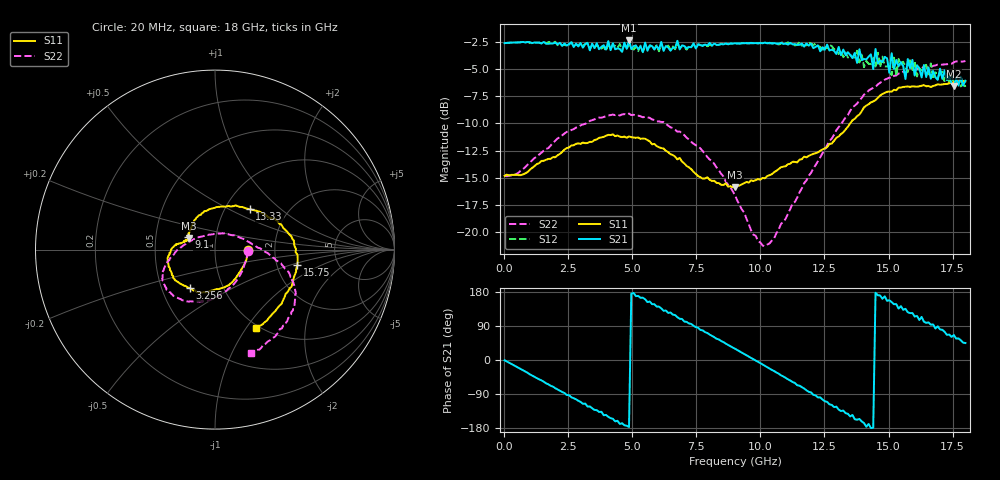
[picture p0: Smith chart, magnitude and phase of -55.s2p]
!Agilent Technologies,N5230A,US43500223,A.07.50.48
!Agilent N5230A: A.07.50.48
!Date: Saturday, January 16, 2016 19:57:11
!Correction: S11(Full 2 Port(1,2))
!S21(Full 2 Port(1,2))
!S12(Full 2 Port(1,2))
!S22(Full 2 Port(1,2))
!S2P File: Measurements: S11, S21, S12, S22:
# Hz S  dB  R 50
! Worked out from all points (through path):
!   201 points, 20 MHz to 18 GHz, reference 50 ohm
!   highest |S21| = -2.38 dB at 4.875 GHz (marker M1); lowest = -6.6 dB at 17.55 GHz (marker M2)
!   group delay of S21, straight-line fit = 105 ps
!   lowest |S11| = -15.9 dB at 9.01 GHz (marker M3), VSWR 1.38, Z = 36.9 + j4.94 ohm
!   |S11| at or under -10 dB: start of sweep to 13.51 GHz
!   |S22| runs from -21.3 to -4.3 dB; largest |S21 - S12| = 0.15
!   S11 on the Smith chart (normalised r, x): 20 MHz: 1.44, -0.01; 3.256 GHz: 0.69, -0.32; 9.1 GHz: 0.74, +0.10; 13.33 GHz: 1.30, +0.64; 15.75 GHz: 2.61, -0.58; 18 GHz: 0.96, -1.11
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2e7  -14.82 -1.6  -2.63 -0.7  -2.62 -0.7  -14.82 -1.9
9.19e8  -14.47 -47.3  -2.52 -33.8  -2.53 -34.1  -13.78 -50.1
1.818e9  -13.26 -81.0  -2.66 -68.1  -2.58 -68.9  -12.02 -82.4
3.0766e9  -11.76 -117.8  -3.04 -115.6  -2.91 -114.9  -10.10 -111.9
3.2564e9  -11.80 -123.5  -2.62 -122.9  -2.59 -122.1  -9.93 -115.4
4.8746e9  -11.20 -160.0  -2.38 -176.7  -2.74 -177.3  -9.10 -140.6
6.0433e9  -12.20 -178.9  -3.20 140.9  -3.38 139.1  -9.82 -155.4
7.3918e9  -14.44 168.7  -2.65 90.3  -2.75 90.8  -11.87 -169.0
9.01e9  -15.89 156.1  -2.65 29.8  -2.67 29.4  -16.60 162.2
9.0999e9  -15.76 155.3  -2.66 26.2  -2.64 25.7  -17.09 158.8
1.05383e10  -14.48 131.5  -2.63 -29.2  -2.74 -30.3  -20.55 71.4
1.20666e10  -12.79 95.0  -3.09 -91.9  -2.81 -90.2  -14.13 11.8
1.33252e10  -10.56 49.2  -3.73 -140.3  -3.47 -139.4  -9.45 -8.6
1.4404e10  -7.98 17.7  -5.01 -178.5  -3.98 179.3  -6.74 -21.6
1.44939e10  -7.86 16.2  -3.16 177.6  -4.78 179.8  -6.64 -21.8
1.50333e10  -7.07 4.3  -5.36 157.8  -4.79 152.2  -5.80 -28.7
1.56626e10  -6.64 -8.9  -5.92 135.1  -4.75 129.8  -5.30 -37.0
1.57525e10  -6.61 -10.7  -4.09 126.0  -5.28 130.5  -5.19 -37.8
1.58424e10  -6.65 -13.4  -4.93 123.7  -4.08 118.7  -5.20 -39.3
1.66515e10  -6.66 -32.1  -5.89 93.3  -4.49 92.9  -4.86 -50.9
1.75505e10  -6.20 -53.7  -6.57 65.8  -6.22 57.0  -4.39 -64.4
1.8e10  -6.13 -62.8  -6.08 44.8  -6.64 43.6  -4.27 -70.8
